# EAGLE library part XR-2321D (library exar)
V.23/V.21 MODEM
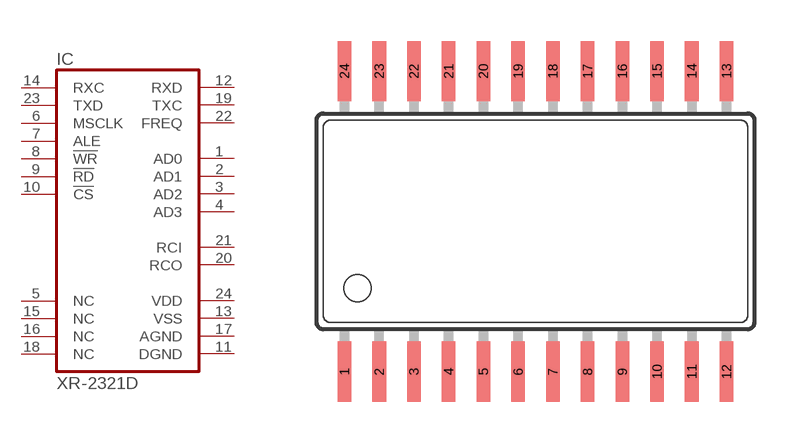
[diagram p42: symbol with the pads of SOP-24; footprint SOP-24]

Designator prefix IC

## XR-2321D (OC_FARNELL: unknown; OC_NEWARK: unknown)  [SOP-24]
1  AD0
2  AD1
3  AD2
4  AD3
5  NC  nc
6  MSCLK  in
7  ALE  in
8  !WR  in
9  !RD  in
10  !CS  in
11  DGND  pwr
12  RXD  out
13  VSS  pwr
14  RXC  in
15  NC  nc
16  NC  nc
17  AGND  pwr
18  NC  nc
19  TXC  out
20  RCO
21  RCI
22  FREQ  out
23  TXD  in
24  VDD  pwr

## Footprint SOP-24 (pad centres in mm)
Small Outline Package
smd 0.5 x 2.2: 1 -6.985,-5.5; 2 -5.715,-5.5; 3 -4.445,-5.5; 4 -3.175,-5.5; 5 -1.905,-5.5; 6 -0.635,-5.5; 7 0.635,-5.5; 8 1.905,-5.5; 9 3.175,-5.5; 10 4.445,-5.5; 11 5.715,-5.5; 12 6.985,-5.5; 13 6.985,5.5; 14 5.715,5.5; 15 4.445,5.5; 16 3.175,5.5; 17 1.905,5.5; 18 0.635,5.5; 19 -0.635,5.5; 20 -1.905,5.5; 21 -3.175,5.5; 22 -4.445,5.5; 23 -5.715,5.5; 24 -6.985,5.5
